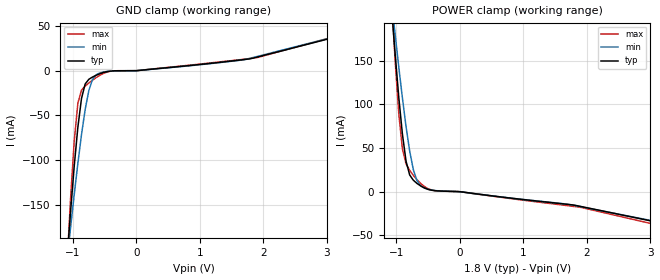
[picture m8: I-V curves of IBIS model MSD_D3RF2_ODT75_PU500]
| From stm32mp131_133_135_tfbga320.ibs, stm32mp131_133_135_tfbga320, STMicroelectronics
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[Model] MSD_D3RF2_ODT75_PU500
Model_type   Input
C_comp 2.322pF   2.256pF   2.387pF
Vinh = 1.150V
Vinl = 650.000mV
[Temperature Range]   25.000   125.000   -40.000
[Voltage Range]   1.800V   1.700V   1.900V
[GND Clamp Reference]   0.00V   0.00V   0.00V
[POWER Clamp Reference]   1.800V   1.700V   1.900V
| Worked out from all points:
|   GND clamp passes 1 mA (typ) near -0.46 V on its own axis
|   POWER clamp passes 1 mA (typ) near -0.38 V on its own axis
[GND Clamp]
-1.785V   -933.7mA   -691.9mA   -1.301A
-1.094V   -212.6mA   -213.2mA   -219.9mA
-1.036V   -157.7mA   -175.3mA   -143.2mA
-978.8mV  -106.9mA   -138.7mA   -78.96mA
-921.2mV  -63.2mA    -103.6mA   -36.44mA
-863.6mV  -31mA      -71.32mA   -21.72mA
-806.1mV  -14.85mA   -43.39mA   -17.19mA
-748.5mV  -9.624mA   -22.18mA   -13.8mA
-633.3mV  -5.128mA   -4.578mA   -7.756mA
-403mV    -416uA     -396uA     -532uA
1.67V     12.21mA    11.98mA    12.61mA
3.57V     45.43mA    45.91mA    46.54mA
[Power Clamp]
-1.77V    940mA      703.9mA    1.301A
-1.079V   213mA      218.8mA    223.5mA
-1.021V   158.4mA    180.5mA    151mA
-963.6mV  108.6mA    143.1mA    89.89mA
-906.1mV  66.12mA    107.4mA    48.98mA
-848.5mV  34.79mA    74.5mA     31.73mA
-790.9mV  19.04mA    46.29mA    24.34mA
-733.3mV  12.98mA    25.14mA    18.6mA
-675.8mV  9.377mA    12.55mA    13.62mA
-560.6mV  4.276mA    4.069mA    5.923mA
1.915V    -17.16mA   -17.44mA   -18.2mA
3.585V    -42.16mA   -41.28mA   -46.16mA
